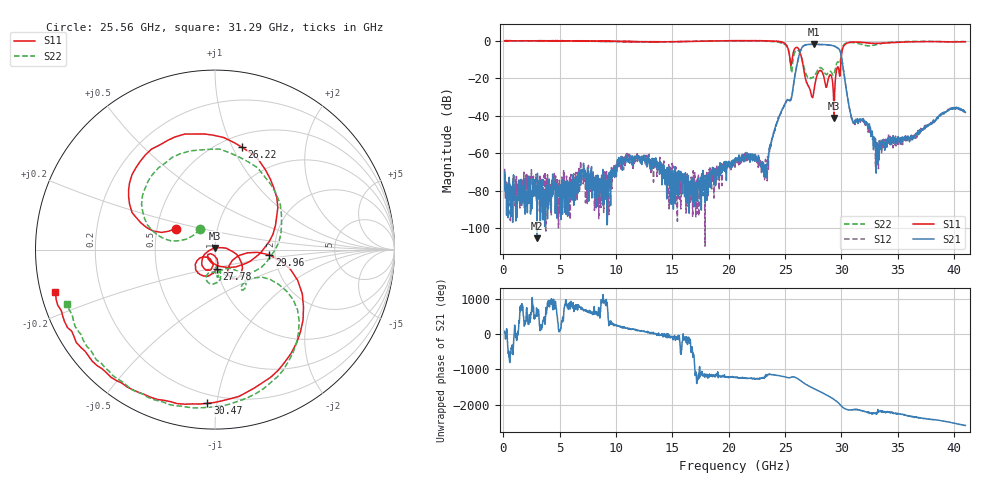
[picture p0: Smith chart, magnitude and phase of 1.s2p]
!The following data was pulled from an Agilent PNA
!This sNp file was generated from the data in the RF Test software
!NOTE:  Smoothing/Math/Corrections applied on any given trace ARE included in the data saved here
# MHz S dB R 50
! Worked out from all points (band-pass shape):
!   1601 points, 100 MHz to 41 GHz, reference 50 ohm
!   highest |S21| = -1.87 dB at 27.58 GHz (marker M1); lowest = -105.4 dB at 2.989 GHz (marker M2)
!   |S21| within 3 dB of the highest: 26.39 GHz to 29.83 GHz (3.443 GHz wide, 12.2 % of centre)
!   lowest |S11| = -41.2 dB at 29.34 GHz (marker M3), VSWR 1.02, Z = 50.1 + j0.872 ohm
!   |S11| at or under -10 dB: 25.43 GHz to 25.61 GHz (179.6 MHz wide, 0.704 % of centre); 26.5 GHz to 29.96 GHz (3.466 GHz wide, 12.3 % of centre)
!   |S22| runs from -20.2 to 0.1 dB; largest |S21 - S12| = 0.01
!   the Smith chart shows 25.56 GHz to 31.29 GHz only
!   S11 on the Smith chart (normalised r, x): 25.56 GHz: 0.63, +0.16; 26.22 GHz: 0.62, +1.09; 27.78 GHz: 1.00, -0.22; 29.96 GHz: 1.86, -0.12; 30.47 GHz: 0.15, -0.94; 31.29 GHz: 0.04, -0.13
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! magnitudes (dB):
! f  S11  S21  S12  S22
! 100 MHz  0.0  -69.9  -68.3  0.0
! 2.989 GHz  -0.1  -105.4  -73.9  0.0
! 6.925 GHz  -0.1  -74.0  -70.0  -0.2
! 9.124 GHz  -0.4  -78.2  -77.3  -0.1
! 10.79 GHz  -0.3  -62.9  -66.6  -0.6
! 13.75 GHz  -0.6  -65.1  -68.0  -0.6
! 17.02 GHz  -0.3  -83.0  -87.2  -0.3
! 20.55 GHz  0.1  -65.3  -67.4  -0.1
! 23.31 GHz  0.0  -69.1  -68.7  -0.3
! 24.18 GHz  -0.2  -45.5  -44.8  -0.5
! 25.56 GHz  -12.1  -30.3  -30.4  -17.1
! 26.22 GHz  -4.6  -8.1  -8.0  -5.6
! 27.38 GHz  -29.9  -1.9  -1.9  -19.8
! 27.58 GHz  -26.0  -1.9  -1.9  -18.8
! 27.78 GHz  -19.3  -1.9  -1.9  -16.9
! 29.34 GHz  -41.2  -2.8  -2.8  -17.8
! 29.96 GHz  -10.3  -7.2  -7.2  -7.9
! 30.47 GHz  -1.3  -27.6  -27.7  -1.1
! 31.29 GHz  -0.7  -42.6  -41.7  -1.1
! 33.25 GHz  -1.4  -56.9  -60.9  -1.9
! 34.2 GHz  -1.1  -52.9  -51.9  -0.9
! 41 GHz  -0.5  -38.2  -38.0  -0.5
